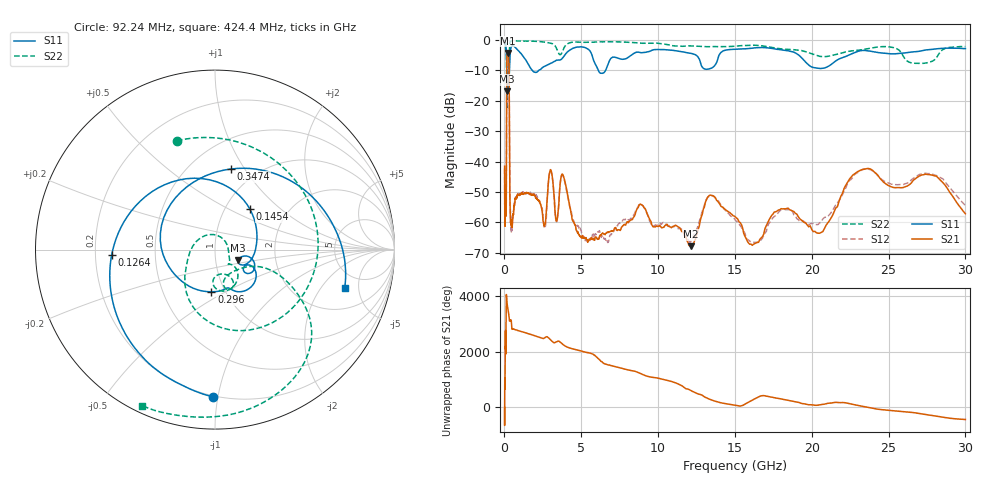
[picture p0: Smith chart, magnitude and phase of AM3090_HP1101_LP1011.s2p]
! Date/Time: Thu, Feb 28, 2019 2:08 PM
! Network Analyzer: Agilent Technologies E8364B Rev: A.07.50.67
! Sweep from 0.010 to 30.000 GHz, 1601 Points, Sweep Type: LOG
! Power Supply: 5.022 V, 0.002 A
# Hz S DB R 50
!freq MagS11 AngS11 MagS21 AngS21 MagS12 AngS12 MagS22 AngS22
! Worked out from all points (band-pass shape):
!   1601 points, 10 MHz to 30 GHz, reference 50 ohm
!   highest |S21| = -4.31 dB at 221.4 MHz (marker M1); lowest = -67.8 dB at 12.13 GHz (marker M2)
!   |S21| within 3 dB of the highest: 152.8 MHz to 288.7 MHz (135.9 MHz wide, 61.6 % of centre)
!   lowest |S11| = -16.9 dB at 174.1 MHz (marker M3), VSWR 1.33, Z = 64.4 - j7.72 ohm
!   |S11| at or under -10 dB: 144.2 MHz to 323.6 MHz (179.4 MHz wide, 76.7 % of centre); 1.813 GHz to 2.236 GHz (423.4 MHz wide, 20.9 % of centre); 6.109 GHz to 6.583 GHz (473.7 MHz wide, 7.46 % of centre)
!   |S22| runs from -22.8 to -0.2 dB; largest |S21 - S12| = 0.016
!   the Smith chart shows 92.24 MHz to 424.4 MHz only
!   S11 on the Smith chart (normalised r, x): 92.24 MHz: 0.19, -0.97; 126.4 MHz: 0.27, -0.02; 145.4 MHz: 1.30, +0.64; 296 MHz: 0.86, -0.43; 347.4 MHz: 0.77, +0.87; 424.4 MHz: 3.50, -3.50
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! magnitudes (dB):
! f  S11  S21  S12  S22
! 10 MHz  -0.3  -41.5  -42.3  -0.6
! 38.04 MHz  -0.4  -59.6  -57.6  -1.5
! 92.24 MHz  -1.7  -55.9  -57.7  -3.8
! 126.4 MHz  -4.8  -41.0  -40.4  -5.3
! 144.7 MHz  -10.2  -11.8  -11.8  -18.9
! 145.4 MHz  -10.5  -11.2  -11.1  -19.7
! 174.1 MHz  -16.9  -4.8  -4.8  -17.6
! 221.4 MHz  -14.5  -4.3  -4.3  -16.0
! 296 MHz  -12.5  -8.8  -8.7  -12.1
! 347.4 MHz  -6.8  -49.6  -50.3  -1.0
! 424.4 MHz  -2.4  -60.0  -61.7  -0.4
! 550.5 MHz  -1.9  -58.7  -57.8  -0.3
! 2.084 GHz  -10.6  -52.2  -51.4  -0.5
! 2.623 GHz  -8.7  -60.9  -61.8  -0.7
! 3.798 GHz  -5.8  -44.3  -44.5  -3.5
! 5.338 GHz  -2.7  -65.7  -65.8  -0.8
! 7.926 GHz  -6.1  -60.4  -58.9  -0.7
! 12.13 GHz  -4.4  -67.8  -66.3  -1.9
! 13.54 GHz  -9.1  -51.2  -51.2  -2.2
! 20.51 GHz  -9.4  -63.6  -60.2  -5.4
! 23.36 GHz  -3.4  -42.6  -42.5  -3.1
! 30 GHz  -2.8  -57.2  -54.5  -2.2
